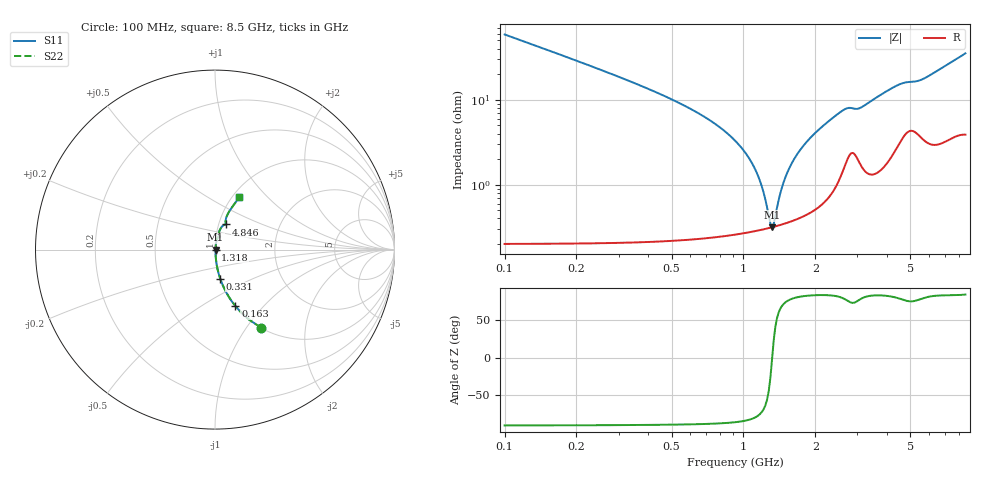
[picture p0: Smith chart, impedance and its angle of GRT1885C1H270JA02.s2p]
!Murata Part Number: GRT1885C1H270JA02
!These Parameters are Measured in Series Mode Connection
!Data Generated on Jun 19, 2026
!  o--ll--o
!Port1  Port2
!  o------o
!Operation Temp=25[degC], DC Bias Voltage=0[V]
!Freq. Start=100[MHz] Stop=9[GHz] 401[Steps]
# Hz S RI R 50
!Freq.(Hz) S11(Real) S11(Imag) S21(Real) S21(Imag) S12(Real) S12(Imag) S22(Real) S22(Imag)
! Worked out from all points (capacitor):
!   401 points, 100 MHz to 8.5 GHz, reference 50 ohm
!   read as one part in series: C = 27 pF near 142 MHz
!   lowest |Z| = 316 mohm at 1.318 GHz (marker M1)
!   series resonance near 1.319 GHz, so ESL is about 540 pH
!   S11 on the Smith chart (normalised r, x): 100 MHz: 1.00, -1.17; 163 MHz: 1.00, -0.71; 331 MHz: 1.00, -0.33; 1.318 GHz: 1.01, -0.00; 4.846 GHz: 1.08, +0.31; 8.5 GHz: 1.08, +0.70
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1e8  0.2564 -0.435  0.7436 0.435  0.7436 0.435  0.2564 -0.435
1.63e8  0.114 -0.315  0.886 0.315  0.886 0.315  0.114 -0.315
3.31e8  0.029 -0.1618  0.971 0.1618  0.971 0.1618  0.029 -0.1618
8.56e8  0.00409 -0.0399  0.9959 0.0399  0.9959 0.0399  0.00409 -0.0399
1.024e9  0.00323 -0.023  0.9968 0.023  0.9968 0.023  0.00323 -0.023
1.15e9  0.00303 -0.0124  0.997 0.0124  0.997 0.0124  0.00303 -0.0124
1.213e9  0.00303 -0.00759  0.997 0.00759  0.997 0.00759  0.00303 -0.00759
1.276e9  0.00308 -0.00302  0.9969 0.00302  0.9969 0.00302  0.00308 -0.00302
1.318e9  0.00314 -9.57e-05  0.9969 9.57e-05  0.9969 9.57e-05  0.00314 -9.57e-05
1.36e9  0.00323 0.00274  0.9968 -0.00274  0.9968 -0.00274  0.00323 0.00274
1.444e9  0.00345 0.0082  0.9966 -0.0082  0.9966 -0.0082  0.00345 0.0082
1.507e9  0.00366 0.0121  0.9963 -0.0121  0.9963 -0.0121  0.00366 0.0121
1.591e9  0.00399 0.0172  0.996 -0.0172  0.996 -0.0172  0.00399 0.0172
1.717e9  0.00462 0.0245  0.9954 -0.0245  0.9954 -0.0245  0.00462 0.0245
2.032e9  0.00696 0.0417  0.993 -0.0417  0.993 -0.0417  0.00696 0.0417
2.599e9  0.019 0.0707  0.981 -0.0707  0.981 -0.0707  0.019 0.0707
2.914e9  0.0276 0.0713  0.9724 -0.0713  0.9724 -0.0713  0.0276 0.0713
4.3e9  0.042 0.1313  0.958 -0.1313  0.958 -0.1313  0.042 0.1313
4.846e9  0.0604 0.1404  0.9396 -0.1404  0.9396 -0.1404  0.0604 0.1404
5.707e9  0.0591 0.1591  0.9409 -0.1591  0.9409 -0.1591  0.0591 0.1591
7.114e9  0.0873 0.2252  0.9127 -0.2252  0.9127 -0.2252  0.0873 0.2252
8.5e9  0.1355 0.2913  0.8645 -0.2913  0.8645 -0.2913  0.1355 0.2913
